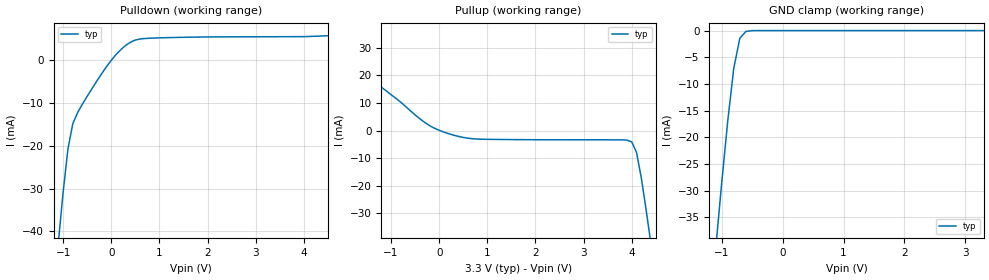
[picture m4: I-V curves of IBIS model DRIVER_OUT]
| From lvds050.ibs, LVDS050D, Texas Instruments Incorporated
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|   Driver Output  MODEL
[Model]   DRIVER_OUT
Model_type   3-state
| Signals   1Y,1Z,2Y,2Z
Vmeas = 1.2V   |Reference voltage for timing measurements
Cref = 5pF   |Timing specification test load capacitance value
Rref = 50   |Note: 50 Ohm load; single ended configuration
Vref = 1.18V   |Timing specification test load voltage
| variable   typ   min   max
C_comp   1.0pF   NA   NA
|   typ   min   max
[Temperature Range]   25.0   NA   NA
[Voltage range]   3.3V   3.0V   3.6V
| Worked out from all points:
|   slope of the pulldown table from 0 to 0.495 V, typ, clamps not added: 105 ohm
|   slope of the pullup table from 0 to 0.495 V, typ, clamps not added: 192 ohm
|   GND clamp passes 1 mA (typ) near -0.67 V on its own axis
[Pulldown]
|   Voltage   I(typ)   I(min)   I(max)
-3.3V     -348mA     NA         NA
-1.1V     -42.6mA    NA         NA
-1V       -30.8mA    NA         NA
-900mV    -20.7mA    NA         NA
-800mV    -14.9mA    NA         NA
-600mV    -10.3mA    NA         NA
-100mV    -1.58mA    NA         NA
200mV     2.42mA     NA         NA
500mV     4.64mA     NA         NA
1.4V      5.26mA     NA         NA
4.1V      5.46mA     NA         NA
6.6V      7.11mA     NA         NA
[Pullup]
|   Voltage   I(typ)   I(min)   I(max)
| Note that the[Pullup]voltage table is referenced to Vcc
| and is calculated using Vtable=Vcc - Vmeasured.
-3.3V     49.3mA     NA         NA
-2.6V     37.7mA     NA         NA
-1.9V     25.6mA     NA         NA
-400mV    4.24mA     NA         NA
200mV     -1.17mA    NA         NA
800mV     -3.11mA    NA         NA
4V        -4.13mA    NA         NA
4.1V      -8.04mA    NA         NA
4.2V      -17.4mA    NA         NA
4.3V      -29mA      NA         NA
4.4V      -41.4mA    NA         NA
6.6V      -348mA     NA         NA
[GND_clamp]
|   Voltage   I(typ)   I(min)   I(max)
| Outputs in High Impedance (off)
-3.3V     -347mA     NA         NA
-1.1V     -41.4mA    NA         NA
-1V       -28.8mA    NA         NA
-900mV    -17.1mA    NA         NA
-800mV    -7.08mA    NA         NA
-700mV    -1.43mA    NA         NA
-600mV    -153uA     NA         NA
-400mV    -866nA     NA         NA
3.3V      -59.7pA    NA         NA
[POWER_clamp]
|   Voltage   I(typ)   I(min)   I(max)
| Note that the [POWER_clamp] voltage table is referenced to Vcc
| and is calculated using Vtable = Vcc - Vmeasured.
| Outputs in Tri-state.
-3.3V     0A         NA         NA
0V        0A         NA         NA
[Ramp]
|   typ   min   max
dV/dt_r   0.201/800ps   NA   NA
dV/dt_f   0.201/800ps   NA   NA
R_load = 100ohm | Note: The measurement is on a differential configuration
